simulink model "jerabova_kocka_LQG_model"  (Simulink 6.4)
settings: Solver=ode45  StartTime=0.0  StopTime=200  RelTol=1e-3
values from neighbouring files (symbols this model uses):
  A = [0 1 0 0 0    [kockaLQG.m]    (also in kockaLQR.m; podklad.m = [dh1_h10 dh1_h20 0; testx.m = [ -0.195 0.195; 0.195 -0.205]; kulicka_na_tyci_LQG_podklad.m = [0 0;1 0])
  B = [0    [kockaLQG.m]    (also in kockaLQR.m; podklad.m = [dh1_q0; testx.m = [0.0047; 0]; kulicka_na_tyci_LQG_podklad.m = [7.14;0])
  C = [1 0 0 0 0]    [kockaLQG.m]    (also in kockaLQR.m; podklad.m = [0 0 1]; testx.m = [0 1]; kulicka_na_tyci_LQG_podklad.m = [0 1])
  D = [0]    [kockaLQG.m]    (also in kockaLQR.m; podklad.m = 0; testx.m; kulicka_na_tyci_LQG_podklad.m = 0)
  K = tf(num,den)    [phinf2.m]
  Ng = lqr_kompenzace(A,B,C,D,K)    [kockaLQG.m]    (also in kockaLQR.m; lqr_kompenzace.m = Nu + K*Nx; testx.m; kulicka_na_tyci_LQG_podklad.m)
undefined symbols (not defined in the file or in its folder): L

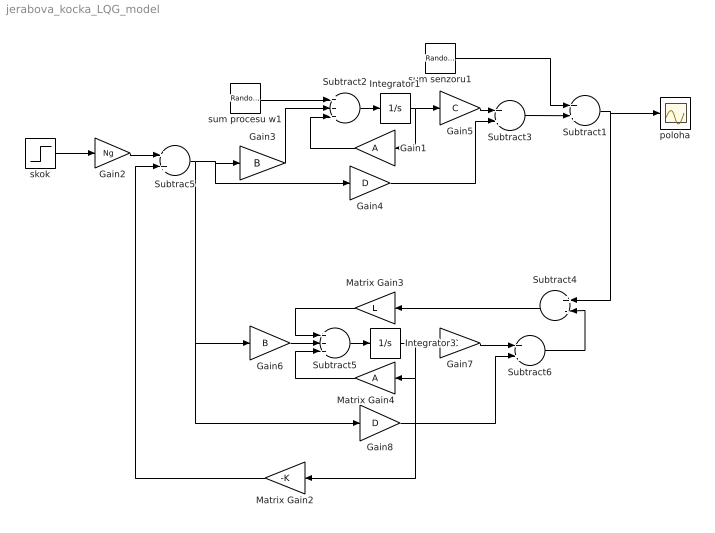
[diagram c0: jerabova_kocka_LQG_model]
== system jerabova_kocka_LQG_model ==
  Gain1 : Gain  Orientation=left  Gain=A  Multiplication=Matrix(K*u)
  Gain2 : Gain  Gain=Ng
  Gain3 : Gain  Gain=B  Multiplication=Matrix(K*u)
  Gain4 : Gain  Gain=D  Multiplication=Matrix(K*u)
  Gain5 : Gain  Gain=C  Multiplication=Matrix(K*u)
  Gain6 : Gain  Gain=B  Multiplication=Matrix(K*u)
  Gain7 : Gain  Gain=C  Multiplication=Matrix(K*u)
  Gain8 : Gain  Gain=D  Multiplication=Matrix(K*u)
  Integrator1 : Integrator
  Integrator3 : Integrator
  Matrix Gain2 : Gain  Orientation=left  Gain=-K  Multiplication=Matrix(K*u)
  Matrix Gain3 : Gain  Orientation=left  Gain=L  Multiplication=Matrix(K*u)
  Matrix Gain4 : Gain  Orientation=left  Gain=A  Multiplication=Matrix(K*u)
  Subtrac5 : Sum  OutScaling=2^-10
  Subtract1 : Sum  OutScaling=2^-10
  Subtract2 : Sum  Inputs=+++  OutScaling=2^-10
  Subtract3 : Sum  OutScaling=2^-10
  Subtract4 : Sum  Orientation=left  Inputs=+-  OutScaling=2^-10
  Subtract5 : Sum  Inputs=+++  OutScaling=2^-10
  Subtract6 : Sum  OutScaling=2^-10
  poloha : Scope
  skok : Step  Time=0  SampleTime=0
  sum procesu w1 : RandomNumber  Variance=0.00002  SampleTime=0
  sum senzoru1 : RandomNumber  Variance=0.00002  SampleTime=0
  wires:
  Integrator1/1 -> Gain5/1, Gain1/1
  Subtract2/1 -> Integrator1/1
  Gain5/1 -> Subtract3/1
  Gain4/1 -> Subtract3/2
  Gain3/1 -> Subtract2/2
  Gain6/1 -> Subtract5/2
  Matrix Gain3/1 -> Subtract5/1
  Subtract4/1 -> Matrix Gain3/1
  Subtract5/1 -> Integrator3/1
  Gain7/1 -> Subtract6/1
  Gain8/1 -> Subtract6/2
  Subtract6/1 -> Subtract4/2
  Matrix Gain4/1 -> Subtract5/3
  Matrix Gain2/1 -> Subtrac5/2
  skok/1 -> Gain2/1
  Subtrac5/1 -> Gain3/1, Gain4/1, Gain6/1, Gain8/1
  Integrator3/1 -> Gain7/1, Matrix Gain4/1, Matrix Gain2/1
  Gain2/1 -> Subtrac5/1
  Subtract3/1 -> Subtract1/2
  Subtract1/1 -> poloha/1, Subtract4/1
  Gain1/1 -> Subtract2/3
  sum senzoru1/1 -> Subtract1/1
  sum procesu w1/1 -> Subtract2/1
